ORGANIZATION_BLOCK MAIN:OB1
TITLE=Ciclo Automatico per due unità operatrici
//Simulatore: 03
//Versione: 1.0
//Data: 15/02/2002
//
//------------- Descrizione del controllo ---------------
// Il programma svolge il controllo di un ciclo automatico
// la cui sequenza operativa prevede:
//
// 1) Ciclo 1 - la prima unità operatrice (motore M1) deve
//    essere avviata a tensione ridotta (Stella/Triangolo)
//    mediante il pulsante SB2 e in seguito arrestata
//    manualmente mediante il pulsante SB1.
// 2) Ciclo 2 - dopo quattro arresti manuali della prima
//    unità deve intervenire automaticamente la seconda
//    unità (motore M2) per un tempo prefissato (10 s)
//    trascorso il quale l'unità si arresta automaticamente.
// 3) Durante il ciclo 2 deve essere impedita l'inserzione
//    della prima unità operatrice.
// 4) L'inserzione della seconda unità può essere eseguita
//    manualmente tramite il pulsante SB3.
//
// Il tempo di commutazione (Y-D) e quello di lavoro della
// seconda unità sono ottenuti mediante due temporizzatori
// software (T33-T34). Per il conteggio delle inserzioni
// consecutive della prima unità è previsto un contatore
// software C0.
// Nel sistema è previsto un arresto di emergenza dovuto
// all'intervento di un circuito di sicurezza esterno simulato
// dal pulsante SB4 il cui intervento porta all'arresto
// delle due unità.
// Ogni unità verrà anche arrestata automaticamente in caso
// di intervento del rispettivo relè termico, il cui intervento
// è previsto via hardware.
// Per ogni unità sono previste due lampade che segnalano
// rispettivamente la marcia del motore, l'arresto.
//

BEGIN
NETWORK 1 //Impostazione bit SCR
//
LD Q0.0
A I0.2
O I0.1
A I0.0
AN Q0.3
A I0.5
= S0.0

NETWORK 2 //Inizio segmento SCR
//
LSCR S0.0

NETWORK 3 //Attivazione Motore M1
//
LD I0.0
= Q0.0

NETWORK 4 //Temporizzatore Stella
//
LDN Q0.2
O Q0.1
TON T33 +50

NETWORK 5 //Attivazione KM2 Stella
//
LDN T33
AN Q0.2
= Q0.1

NETWORK 6 //Gestione Fase Triangolo Motore M1
//
LD T33
O Q0.2
AN Q0.1
= Q0.2

NETWORK 7 //Fine segmento SCR
//
SCRE

NETWORK 8 //Contatore cicli Motore M1
//
LD Q0.2
ED
LD T34
CTU C0 +4

NETWORK 9 //Marcia Motore M2
//
LD Q0.3
A I0.4
O I0.3
O C0
AN T34
A I0.5
= Q0.3

NETWORK 10 //Temporizzatore Marcia Motore M2
//
LD Q0.3
TON T34 +100

NETWORK 11 //Segnalazione Arresto Motore M1
//
LDN Q0.0
= Q0.4

NETWORK 12 //Segnalazione Marcia Motore M1
//
LD Q0.1
O Q0.2
= Q0.5

NETWORK 13 //Segnalazione Arresto Motore M2
//
LDN Q0.3
= Q0.6

NETWORK 14 //Segnalazione Marcia Motore M2
//
LD Q0.3
= Q0.7

END_ORGANIZATION_BLOCK

